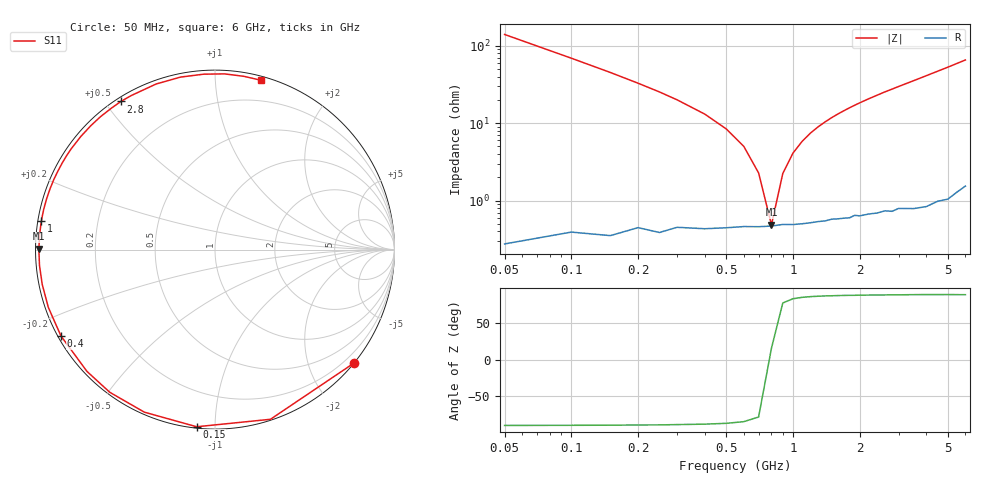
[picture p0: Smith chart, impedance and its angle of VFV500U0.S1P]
! Infineon Technologies  Discrete & RF Semiconductors
! BBY 58-03
! Si Tuning Diode in SOD323
! VR = 0.5 V
! S-Parameters:  June  1999
# GHz  S  MA  R  50
!  f  S11
! GHz  MAG  ANG
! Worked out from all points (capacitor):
!   34 points, 50 MHz to 6 GHz, reference 50 ohm
!   read as one part to ground: C = 22.7 pF near 50 MHz
!   lowest |Z| = 486 mohm at 800 MHz (marker M1)
!   series resonance near 794.4 MHz, so ESL is about 1.8 nH
!   S11 on the Smith chart (normalised r, x): 50 MHz: 0.01, -2.79; 150 MHz: 0.01, -0.90; 400 MHz: 0.01, -0.26; 1 GHz: 0.01, +0.08; 2.8 GHz: 0.01, +0.55; 6 GHz: 0.03, +1.31
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0.05  0.9988 -39.4
0.1  0.9946 -71.9
0.15  0.9923 -95.9
0.2  0.9876 -113.5
0.25  0.9878 -126.4
0.3  0.9846 -136.4
0.4  0.9839 -150.7
0.5  0.9828 -160.9
0.6  0.9819 -168.6
0.7  0.9818 -174.9
0.8  0.9815 179.7
1  0.9807 170.7
1.2  0.98 163.1
1.3  0.9795 159.7
1.6  0.9785 150.5
1.8  0.9785 145.0
2  0.9779 139.9
2.2  0.9774 135.1
2.4  0.9775 130.7
2.6  0.9768 126.3
2.8  0.9779 122.4
3  0.9769 118.5
3.5  0.9792 109.6
4  0.9802 101.3
4.5  0.9794 93.7
5  0.9805 86.9
5.5  0.9788 80.5
6  0.9776 74.8
